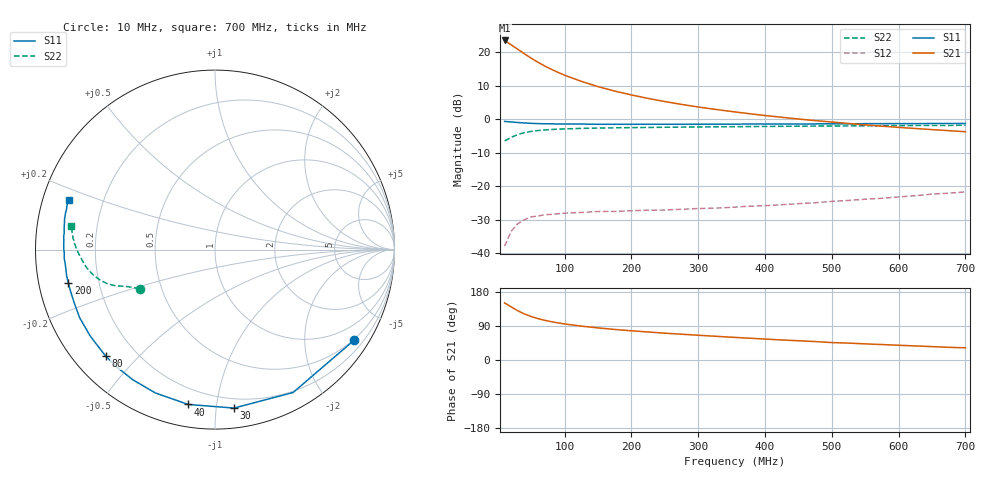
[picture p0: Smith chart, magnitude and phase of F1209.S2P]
! Date: Fri Aug 11 10:42:05 1995
# MHZ  S  MA  R  50.0000
!  POLYFET RF DEVICES
!  F1209 (Each Side)
!  S PARAMETERS
!  VDS=12.5V, IDQ=200mA
!FREQ  S11MAG S11ANG S21MAG S21ANG S12MAG S12ANG S22MAG S22ANG
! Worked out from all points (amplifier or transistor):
!   34 points, 10 MHz to 700 MHz, reference 50 ohm
!   highest |S21| = 23.5 dB at 10 MHz (marker M1)
!   |S21| within 3 dB of that: start of sweep to 32.44 MHz
!   unconditionally stable (mu >= 1): 347.8 MHz to end of sweep
!   at 60 MHz: K = 0.21, MSG = 22.9 dB, |S12| = -28.9 dB
!   at 300 MHz: K = 0.89, MSG = 15.1 dB, |S12| = -26.7 dB
!   at 700 MHz: K = 1.05, MAG = 7.5 dB, |S12| = -21.7 dB
!   S11 on the Smith chart (normalised r, x): 10 MHz: 0.47, -3.30; 30 MHz: 0.13, -1.12; 40 MHz: 0.11, -0.84; 80 MHz: 0.09, -0.40; 200 MHz: 0.09, -0.11; 700 MHz: 0.08, +0.17
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10  0.9248 -33.1  14.91 150.6  0.01273 64.0  0.4731 -152.7
20  0.9072 -61.3  12.81 140.0  0.02138 53.6  0.5347 -157.4
30  0.8892 -83.2  10.96 129.7  0.02769 45.9  0.59 -160.0
40  0.8757 -99.8  9.384 121.2  0.03172 39.7  0.6295 -162.4
50  0.8651 -112.5  8.09 114.6  0.03487 34.9  0.6562 -164.7
60  0.8577 -122.3  7.052 109.2  0.0359 31.6  0.6757 -166.5
70  0.853 -130.0  6.208 104.8  0.0375 29.6  0.6896 -168.0
80  0.8502 -135.8  5.539 101.1  0.03793 27.2  0.7001 -169.1
90  0.845 -141.1  4.982 98.0  0.03875 26.4  0.7085 -170.2
100  0.8458 -145.2  4.517 95.1  0.03962 25.4  0.7154 -171.1
125  0.8443 -153.3  3.656 89.3  0.04053 23.9  0.7272 -172.8
150  0.8386 -159.2  3.051 84.7  0.04189 23.6  0.7352 -174.2
175  0.8376 -163.5  2.617 80.6  0.04194 23.9  0.7418 -175.3
200  0.8378 -167.1  2.293 77.1  0.04304 24.1  0.7469 -176.2
225  0.8393 -170.0  2.035 73.9  0.0438 25.1  0.751 -177.0
250  0.8379 -172.6  1.828 70.8  0.04412 26.4  0.7557 -177.7
300  0.8418 -176.7  1.516 65.3  0.04641 28.7  0.7636 -179.0
375  0.8436 178.2  1.21 57.7  0.05014 33.6  0.7741 179.3
425  0.8464 175.1  1.065 52.8  0.05288 36.5  0.7808 178.0
475  0.8482 172.4  0.9504 48.7  0.05658 39.1  0.7868 176.8
600  0.8576 165.9  0.753 38.9  0.06904 44.3  0.7992 173.5
700  0.861 161.1  0.6483 32.2  0.08222 46.1  0.8114 170.6
